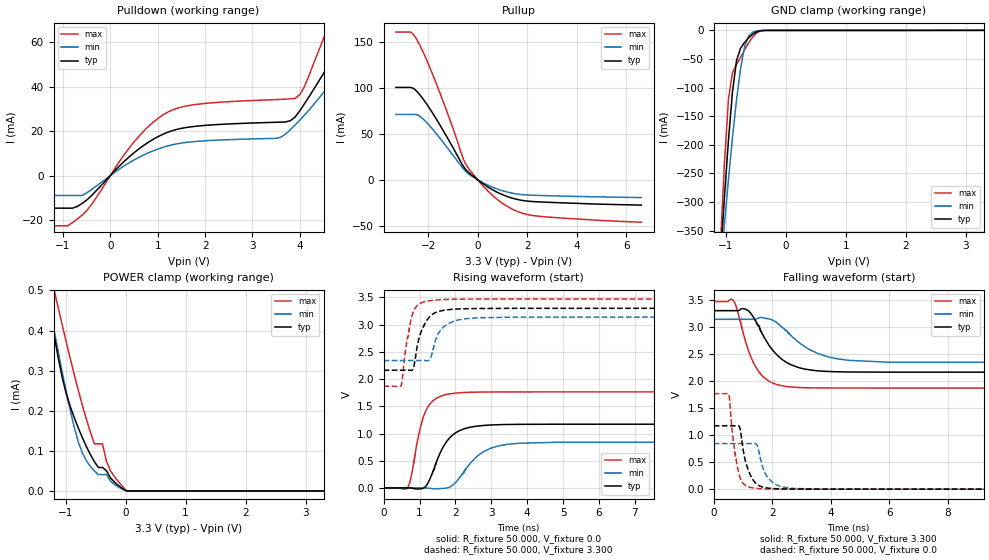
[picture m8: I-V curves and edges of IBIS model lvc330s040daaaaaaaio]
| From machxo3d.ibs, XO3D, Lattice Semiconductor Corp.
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|   Model lvc330s040daaaaaaaio
[Model] lvc330s040daaaaaaaio
Model_type I/O
Polarity   Non-Inverting
Enable   Active-Low
Vinl =  0.800V
Vinh =  2.000V
Vmeas =  1.650V
Cref =  0.0F
Rref =  1.000M
Vref =  0.0V
C_comp   4.200pF   3.800pF   7.500pF
[Temperature Range]   25.000   0.105k   -40.000
[Voltage Range]   3.300V   3.140V   3.470V
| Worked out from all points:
|   slope of the pulldown table from 0 to 0.495 V, typ, clamps not added: 48.6 ohm
|   slope of the pullup table from 0 to 0.495 V, typ, clamps not added: 53.4 ohm
|   GND clamp passes 1 mA (typ) near -0.43 V on its own axis
|   POWER clamp passes 1 mA (typ) near -1.85 V on its own axis
|   rising waveform, R_fixture 50.000, V_fixture 0.0: 20-80 % time 531ps typ, 712ps min, 364ps max; typ from 0 V to 1.17 V
|   rising waveform, R_fixture 50.000, V_fixture 3.300: 20-80 % time 314ps typ, 356ps min, 236ps max; typ from 2.16 V to 3.3 V
|   falling waveform, R_fixture 50.000, V_fixture 3.300: 20-80 % time 887ps typ, 1.24ns min, 634ps max; typ from 3.3 V to 2.16 V
|   falling waveform, R_fixture 50.000, V_fixture 0.0: 20-80 % time 319ps typ, 373ps min, 254ps max; typ from 1.17 V to 0 V
[Pulldown]
|Voltage   I(typ)   I(min)   I(max)
-3.3V     -14.66mA   -8.951mA   -22.6mA
-900mV    -14.66mA   -8.951mA   -22.6mA
-600mV    -12.62mA   -8.951mA   -17.88mA
500mV     10.27mA    7.01mA     15.14mA
1.1V      18.49mA    12.63mA    27.15mA
1.8V      22.18mA    15.35mA    31.97mA
3.6V      24.04mA    17.29mA    34.28mA
4V        29.15mA    24.94mA    36.43mA
4.6V      49.5mA     40.11mA    67.13mA
5V        64.78mA    51.73mA    90.47mA
5.5V      86.24mA    67.68mA    123.5mA
6.6V      140mA      105.9mA    207.2mA
[Pullup]
|Voltage   I(typ)   I(min)   I(max)
-3.3V     100.7mA    71.26mA    161mA
-2.7V     100.7mA    71.26mA    161mA
-2.5V     97.56mA    71.26mA    154.8mA
-2.2V     87.92mA    66.12mA    139mA
-1.7V     67.5mA     51.18mA    106.8mA
-1.2V     44.66mA    33.97mA    71.11mA
-500mV    11.69mA    9.496mA    17.83mA
200mV     -4.043mA   -3.026mA   -6.275mA
800mV     -13.76mA   -10.18mA   -21.62mA
1.5V      -20.8mA    -15.09mA   -33.3mA
2.2V      -23.66mA   -16.79mA   -38.85mA
6.6V      -27.59mA   -19.35mA   -46.21mA
[GND_clamp]
|Voltage   I(typ)   I(min)   I(max)
-3.3V     -4.507A    -3.482A    -6.263A
-1.089V   -398.4mA   -420.6mA   -374.7mA
-1.022V   -290.7mA   -338.6mA   -230.6mA
-955mV    -191.4mA   -260.2mA   -120.1mA
-888mV    -107.5mA   -187mA     -73.7mA
-821mV    -53mA      -121.4mA   -59.85mA
-754mV    -31.41mA   -66.94mA   -47.47mA
-687mV    -21.17mA   -28.82mA   -34.25mA
-620mV    -13.21mA   -10.23mA   -22mA
-553mV    -6.875mA   -3.578mA   -11.73mA
-352mV    -176.3uA   -89.98uA   -279uA
3.3V      50.87nA    0A         -26.43uA
[POWER_clamp]
|Voltage   I(typ)   I(min)   I(max)
-3.3V     3.967mA    2.512mA    11.53mA
-1.323V   507.3uA    506.4uA    605.6uA
-1.256V   446.6uA    452.8uA    548.7uA
-1.189V   387.7uA    399.8uA    501.1uA
-988mV    242.5uA    247.5uA    371.4uA
-854mV    182.6uA    158.2uA    289.7uA
-720mV    133.1uA    94.82uA    213.9uA
-519mV    73.06uA    49.89uA    117.5uA
-385mV    58.36uA    40.66uA    117.5uA
-251mV    32.53uA    24.74uA    49.87uA
-50mV     5.761uA    3.987uA    11.09uA
3.3V      0A         0A         0A
[Ramp]
| variable   typ   min   max
dV/dt_r   0.703/0.532n   0.506/0.719n   1.059/0.365n
dV/dt_f   0.682/0.894n   0.480/1.224n   0.960/0.631n
R_load = 50.000
[Rising Waveform]
R_fixture= 50.000
V_fixture= 0.0
V_fixture_min= 0.0
V_fixture_max= 0.0
|time   V(typ)   V(min)   V(max)
0s        27.06nV    64.78nV    334.4nV
686ps     555uV      -1.899uV   21.47mV
767ps     -1.047mV   -1.899uV   207.2mV
983ps     -18.56mV   119.4uV    998.7mV
1.189ns   41.81mV    41.04uV    1.435V
1.663ns   758.2mV    -9.15mV    1.702V
1.956ns   990mV      68.94mV    1.739V
2.805ns   1.149V     674.3mV    1.762V
3.762ns   1.169V     820.9mV    1.764V
20ns      1.171V     842.7mV    1.765V
[Rising Waveform]
R_fixture= 50.000
V_fixture= 3.300
V_fixture_min= 3.140
V_fixture_max= 3.470
|time   V(typ)   V(min)   V(max)
0s        2.163V     2.341V     1.87V
489ps     2.163V     2.341V     1.883V
636ps     2.163V     2.341V     2.65V
799ps     2.165V     2.341V     3.179V
1.028ns   2.842V     2.341V     3.394V
1.26ns    3.129V     2.343V     3.438V
1.37ns    3.195V     2.526V     3.448V
1.666ns   3.263V     2.957V     3.461V
2.68ns    3.297V     3.127V     3.47V
20ns      3.3V       3.14V      3.47V
[Falling Waveform]
R_fixture= 50.000
V_fixture= 3.300
V_fixture_min= 3.140
V_fixture_max= 3.470
|time   V(typ)   V(min)   V(max)
0s        3.3V       3.14V      3.47V
659ps     3.299V     3.14V      3.497V
811ps     3.299V     3.14V      3.296V
1.186ns   3.298V     3.139V     2.562V
1.68ns    2.856V     3.168V     2.082V
2.055ns   2.543V     3.114V     1.953V
2.433ns   2.363V     2.944V     1.901V
3.311ns   2.202V     2.57V      1.873V
4.617ns   2.166V     2.381V     1.87V
20ns      2.163V     2.341V     1.87V
[Falling Waveform]
R_fixture= 50.000
V_fixture= 0.0
V_fixture_min= 0.0
V_fixture_max= 0.0
|time   V(typ)   V(min)   V(max)
0s        1.171V     842.7mV    1.765V
516ps     1.171V     842.6mV    1.749V
647ps     1.171V     842.7mV    985.1mV
857ps     1.171V     842.7mV    288.2mV
1.094ns   495.7mV    842.5mV    65.29mV
1.336ns   175.4mV    843.5mV    22.81mV
1.485ns   87.81mV    808.3mV    12.9mV
1.881ns   18.74mV    191.9mV    3.431mV
2.782ns   1.671mV    11.75mV    256.6uV
20ns      32.05nV    128nV      313.9nV
